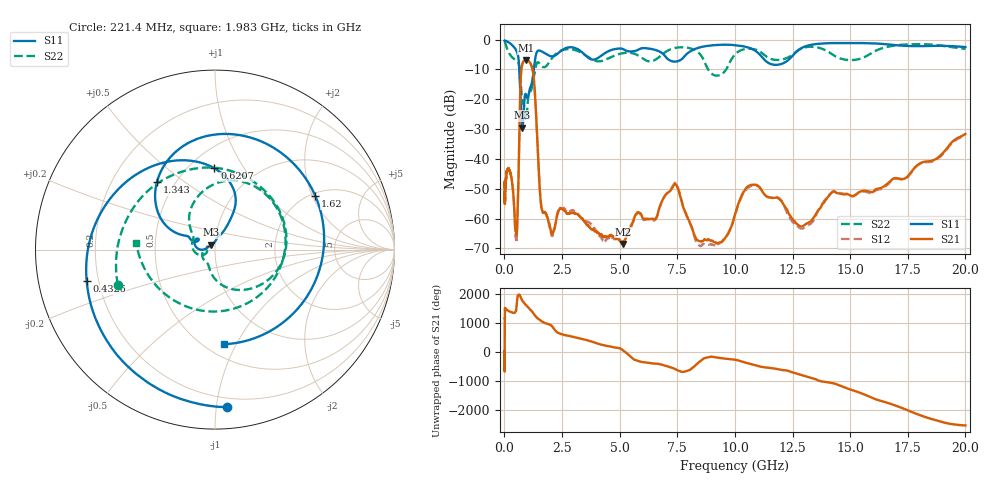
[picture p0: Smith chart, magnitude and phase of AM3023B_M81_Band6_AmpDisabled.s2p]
!Agilent Technologies,E8364B,MY43040894,A.07.50.67
!Agilent E8364B: A.07.50.67
!Date: Tuesday, October 27, 2020 10:38:33
!Correction: S11(Full 2 Port(1,2))
!S21(Full 2 Port(1,2))
!S12(Full 2 Port(1,2))
!S22(Full 2 Port(1,2))
!S2P File: Measurements: S11, S21, S12, S22:Log Frequency Sweep
# Hz S  dB  R 50
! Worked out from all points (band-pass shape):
!   3201 points, 10 MHz to 20 GHz, reference 50 ohm
!   highest |S21| = -6.89 dB at 933.9 MHz (marker M1); lowest = -68.5 dB at 5.14 GHz (marker M2)
!   |S21| within 3 dB of the highest: 738.7 MHz to 1.216 GHz (477.6 MHz wide, 48.9 % of centre)
!   lowest |S11| = -29.5 dB at 783.4 MHz (marker M3), VSWR 1.07, Z = 48 + j2.59 ohm
!   |S11| at or under -10 dB: 643.5 MHz to 1.274 GHz (630.9 MHz wide, 65.8 % of centre)
!   |S22| runs from -26.9 to -0.7 dB; largest |S21 - S12| = 0.0078
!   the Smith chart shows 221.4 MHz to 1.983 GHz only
!   S11 on the Smith chart (normalised r, x): 221.4 MHz: 0.14, -1.07; 432.6 MHz: 0.15, -0.12; 620.7 MHz: 0.66, +0.75; 1.343 GHz: 0.40, +0.40; 1.62 GHz: 2.10, +2.11; 1.983 GHz: 0.61, -0.89
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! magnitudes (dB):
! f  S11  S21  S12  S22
! 10 MHz  -0.3  -49.4  -47.6  -0.7
! 35.55 MHz  -0.4  -51.4  -51.1  -1.0
! 126.1 MHz  -0.7  -43.8  -43.7  -3.2
! 221.4 MHz  -1.1  -43.9  -43.8  -4.8
! 432.6 MHz  -2.7  -57.5  -57.7  -6.6
! 447.2 MHz  -2.8  -59.4  -60.0  -6.7
! 531.9 MHz  -3.9  -65.2  -67.2  -7.2
! 620.7 MHz  -6.9  -43.8  -44.0  -8.0
! 697.3 MHz  -19.4  -15.0  -15.1  -12.9
! 783.4 MHz  -29.5  -8.1  -8.1  -21.0
! 933.9 MHz  -18.3  -6.9  -7.0  -26.9
! 1.343 GHz  -6.1  -20.3  -20.4  -9.8
! 1.59 GHz  -3.9  -55.2  -55.3  -8.6
! 1.62 GHz  -4.0  -56.8  -56.7  -8.9
! 1.983 GHz  -5.5  -62.9  -63.8  -7.1
! 5.14 GHz  -3.1  -68.5  -67.7  -4.5
! 5.639 GHz  -3.9  -59.6  -60.0  -4.8
! 7.358 GHz  -7.4  -48.6  -48.3  -2.9
! 9.09 GHz  -1.9  -67.9  -68.9  -11.9
! 10.81 GHz  -3.4  -48.6  -48.8  -3.2
! 12.98 GHz  -2.5  -62.4  -63.3  -2.7
! 20 GHz  -2.5  -31.6  -32.0  -3.1
